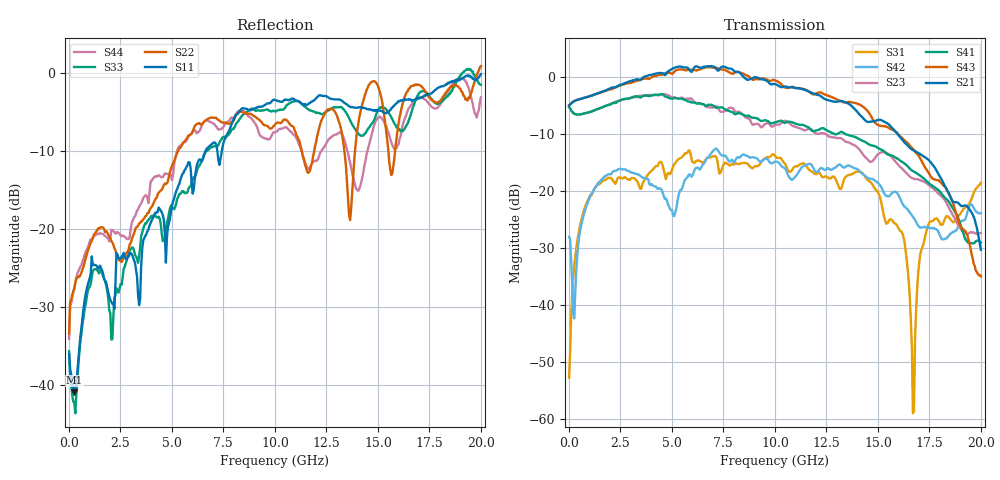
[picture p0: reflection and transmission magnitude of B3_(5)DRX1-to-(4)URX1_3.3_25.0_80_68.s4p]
!Agilent Technologies,N5225A,MY51451112,A.09.50.13
!Agilent N5225A: A.09.50.13
!Date: Sunday, March 12, 2017 05:21:24
!Correction: S11(Full 4 Port(1,2,3,4))
!S12(Full 4 Port(1,2,3,4))
!S13(Full 4 Port(1,2,3,4))
!S14(Full 4 Port(1,2,3,4))
!S21(Full 4 Port(1,2,3,4))
!S22(Full 4 Port(1,2,3,4))
!S23(Full 4 Port(1,2,3,4))
!S24(Full 4 Port(1,2,3,4))
!S31(Full 4 Port(1,2,3,4))
!S32(Full 4 Port(1,2,3,4))
!S33(Full 4 Port(1,2,3,4))
!S34(Full 4 Port(1,2,3,4))
!S41(Full 4 Port(1,2,3,4))
!S42(Full 4 Port(1,2,3,4))
!S43(Full 4 Port(1,2,3,4))
!S44(Full 4 Port(1,2,3,4))
!S4P File: Measurements: <S11,S12,S13,S14>,
!<S21,S22,S23,S24>,
!<S31,S32,S33,S34>,
!<S41,S42,S43,S44>:
# Hz S  dB  R 50
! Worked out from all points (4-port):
!   401 points, 10 MHz to 20 GHz, reference 50 ohm
!   strongest paths, dB at 10 MHz, 5.008 GHz, 10.01 GHz, 15 GHz, 20 GHz:
!     S21: -5.0, 1.4, -1.3, -7.6, -30.4
!     S43: -5.0, 0.5, -0.6, -8.4, -35.0
!     S41: -5.3, -3.9, -8.0, -12.5, -29.1
!     S23: -5.3, -3.6, -8.5, -13.6, -27.4
!     S42: -28.1, -23.4, -14.9, -18.6, -23.9
!     S31: -52.8, -16.3, -13.9, -20.3, -18.6
!   lowest |S11| = -41.0 dB at 259.9 MHz (marker M1), VSWR 1.02, Z = 50.3 - j0.861 ohm
!   |S11| at or under -10 dB: start of sweep to 6.639 GHz; 7.204 GHz to 7.425 GHz (220.2 MHz wide, 3.01 % of centre)
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1e7  -36.01 -37.9  -63.96 -157.9  -52.49 18.1  -62.64 175.5
     -5.02 1.4  -33.45 38.9  -5.33 180.0  -28.04 37.9
     -52.81 17.3  -76.05 82.6  -35.70 -45.7  -65.66 138.5
     -5.34 -180.0  -28.08 38.3  -5.00 1.5  -34.12 45.2
2.59875e8  -40.97 -73.2  -49.93 55.0  -33.19 94.9  -50.85 49.8
           -4.28 -3.5  -27.67 -131.6  -6.47 168.0  -42.00 -161.4
           -33.19 95.1  -49.72 57.3  -42.22 -79.7  -50.57 55.1
           -6.47 167.2  -42.41 -170.9  -4.26 -4.3  -27.71 -137.6
5.2074e9  -15.18 85.9  -35.96 11.0  -15.08 29.7  -37.54 -4.5
          1.68 172.1  -10.63 142.4  -3.76 -29.9  -23.66 65.2
          -14.88 27.5  -36.39 8.5  -16.75 103.1  -42.81 -21.7
          -3.73 -46.2  -23.28 65.6  1.14 162.2  -10.50 120.6
8.30585e9  -4.84 37.3  -39.56 -99.3  -15.41 -1.1  -36.59 -139.6
           0.67 19.8  -4.96 79.5  -6.23 -160.6  -13.85 46.7
           -15.27 -1.8  -32.61 -124.1  -5.86 57.3  -32.04 -161.9
           -6.42 176.2  -14.17 50.6  0.74 7.3  -4.81 45.0
1.22039e10  -2.88 -18.9  -33.94 -155.8  -16.73 -23.2  -35.35 164.3
            -3.34 -145.3  -6.54 68.2  -9.92 40.2  -15.93 38.9
            -17.07 -22.2  -34.15 -145.3  -5.23 -6.1  -33.07 170.3
            -9.17 3.6  -16.09 41.9  -2.74 -170.0  -10.23 -6.8
1.670165e10  -3.55 -75.8  -34.84 117.7  -49.13 -12.7  -36.60 85.9
             -12.87 17.3  -1.63 65.9  -17.85 174.3  -24.75 57.3
             -59.06 -37.1  -33.12 121.9  -4.44 -82.4  -33.14 84.1
             -16.54 122.5  -24.60 57.4  -12.68 -32.8  -3.70 -61.2
2e10  -0.18 -114.1  -33.00 63.2  -18.63 121.4  -35.51 21.2
      -30.36 -136.8  0.84 17.1  -27.42 37.3  -23.91 101.8
      -18.61 121.4  -33.95 39.9  -1.54 -87.6  -35.25 -7.8
      -29.10 -5.5  -23.93 102.8  -35.03 -161.8  -3.18 -136.5
